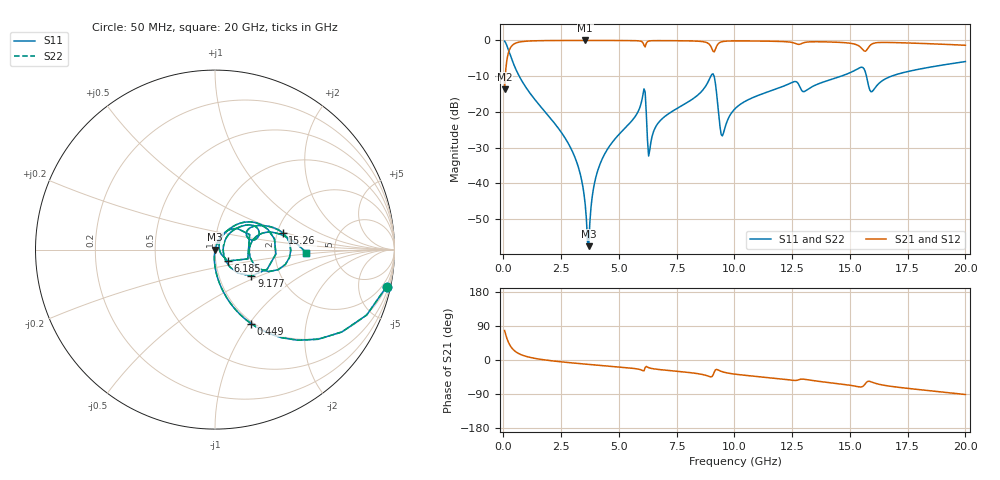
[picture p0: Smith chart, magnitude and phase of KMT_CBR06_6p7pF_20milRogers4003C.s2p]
! Data measured by Modelithics Inc. support@modelithics.com 813-866-6335
! KEMET CBR0603 6.7pF, Pad Width= 0.851mm, Pad Length= 0.64mm, Pad Gap= 0.62mm, 20mil Rogers 4003C substrate Data, January 2022
# hz S ma R 50
! 2 Port Network Data from SP1.SP block
! freq  magS11  angS11  magS21  angS21  magS12  angS12  magS22  angS22
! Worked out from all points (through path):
!   401 points, 50 MHz to 20 GHz, reference 50 ohm
!   highest |S21| = -0.01 dB at 3.541 GHz (marker M1); lowest = -13.6 dB at 50 MHz (marker M2)
!   group delay of S21, straight-line fit = 14 ps
!   lowest |S11| = -57.6 dB at 3.691 GHz (marker M3), VSWR 1.00, Z = 50.1 + j0.0546 ohm
!   |S11| at or under -10 dB: 682.9 MHz to 8.979 GHz (8.296 GHz wide, 172 % of centre); 9.117 GHz to 14.62 GHz (5.505 GHz wide, 46.4 % of centre); 15.72 GHz to 16.8 GHz (1.084 GHz wide, 6.66 % of centre)
!   |S22| runs from -57.6 to -0.2 dB; largest |S21 - S12| = 0
!   S11 on the Smith chart (normalised r, x): 50 MHz: 0.98, -9.29; 449 MHz: 0.98, -1.02; 6.185 GHz: 1.14, -0.15; 9.177 GHz: 1.43, -0.44; 15.26 GHz: 2.14, +0.47; 20 GHz: 3.04, -0.13
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5e7  0.9781 -12.2  0.2079 77.8  0.2079 77.8  0.9781 -12.2
2.495e8  0.6843 -47.6  0.7287 42.4  0.7287 42.4  0.6843 -47.6
4.49e8  0.4589 -64.0  0.888 25.9  0.888 25.9  0.4589 -64.0
2.74325e9  0.03929 -95.0  0.9982 -6.3  0.9982 -6.3  0.03929 -95.0
3.391625e9  0.01082 -94.6  0.9988 -10.0  0.9988 -10.0  0.01082 -94.6
3.54125e9  0.005017 -88.8  0.9988 -10.8  0.9988 -10.8  0.005017 -88.8
3.690875e9  0.00132 24.4  0.9988 -11.6  0.9988 -11.6  0.00132 24.4
3.990125e9  0.0118 71.4  0.9987 -13.2  0.9987 -13.2  0.0118 71.4
4.389125e9  0.02597 72.1  0.9983 -15.2  0.9983 -15.2  0.02597 72.1
6.035e9  0.1704 44.0  0.9343 -28.2  0.9343 -28.2  0.1704 44.0
6.184625e9  0.09527 -41.8  0.9125 -17.0  0.9125 -17.0  0.09527 -41.8
6.33425e9  0.02916 39.9  0.9854 -21.2  0.9854 -21.2  0.02916 39.9
6.73325e9  0.07204 62.1  0.9936 -25.1  0.9936 -25.1  0.07204 62.1
8.828e9  0.2511 37.9  0.9235 -41.7  0.9235 -41.7  0.2511 37.9
9.177125e9  0.2499 -35.7  0.7524 -26.1  0.7524 -26.1  0.2499 -35.7
9.476375e9  0.04608 5.4  0.9622 -30.9  0.9622 -30.9  0.04608 5.4
1.0025e10  0.1106 47.8  0.9843 -37.4  0.9843 -37.4  0.1106 47.8
1.336662e10  0.2253 31.8  0.9577 -54.1  0.9577 -54.1  0.2253 31.8
1.526188e10  0.3888 13.8  0.876 -69.5  0.876 -69.5  0.3888 13.8
1.596012e10  0.1927 2.9  0.8929 -58.6  0.8929 -58.6  0.1927 2.9
1.670825e10  0.3078 18.3  0.9362 -68.9  0.9362 -68.9  0.3078 18.3
2e10  0.5059 -1.8  0.8547 -91.0  0.8547 -91.0  0.5059 -1.8
